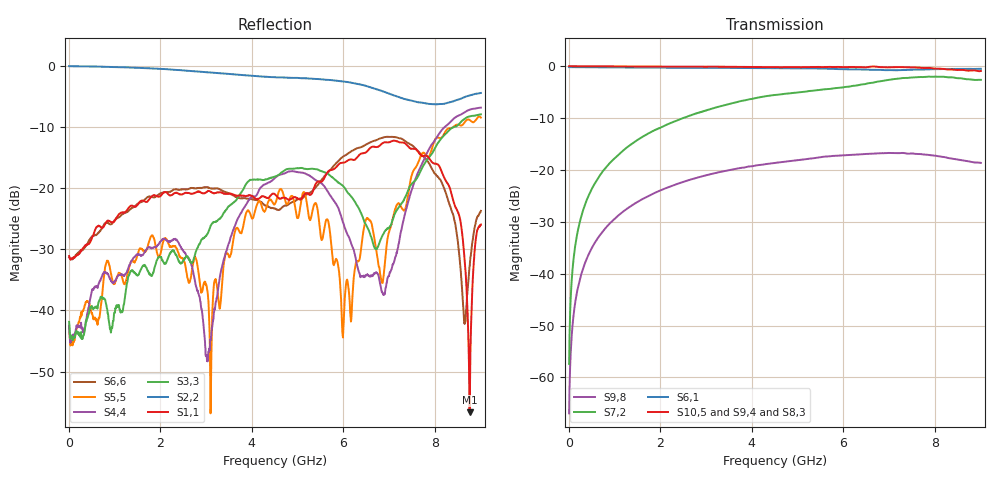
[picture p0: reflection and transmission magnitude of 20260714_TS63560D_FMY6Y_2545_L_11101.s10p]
# GHz S DB R 50
! CMT, SN0916, 25263762, 26.7.0
! Date: 15.07.2026 13:50:19
! Data: Format
! Freq S1.1:dB/Ang S1.2:dB/Ang S1.3:dB/Ang S1.4:dB/Ang S1.5:dB/Ang S1.6:dB/Ang S1.7:dB/Ang S1.8:dB/Ang S1.9:dB/Ang S1.10:dB/Ang
!  S2.1:dB/Ang S2.2:dB/Ang S2.3:dB/Ang S2.4:dB/Ang S2.5:dB/Ang S2.6:dB/Ang S2.7:dB/Ang S2.8:dB/Ang S2.9:dB/Ang S2.10:dB/Ang
!  S3.1:dB/Ang S3.2:dB/Ang S3.3:dB/Ang S3.4:dB/Ang S3.5:dB/Ang S3.6:dB/Ang S3.7:dB/Ang S3.8:dB/Ang S3.9:dB/Ang S3.10:dB/Ang
!  S4.1:dB/Ang S4.2:dB/Ang S4.3:dB/Ang S4.4:dB/Ang S4.5:dB/Ang S4.6:dB/Ang S4.7:dB/Ang S4.8:dB/Ang S4.9:dB/Ang S4.10:dB/Ang
!  S5.1:dB/Ang S5.2:dB/Ang S5.3:dB/Ang S5.4:dB/Ang S5.5:dB/Ang S5.6:dB/Ang S5.7:dB/Ang S5.8:dB/Ang S5.9:dB/Ang S5.10:dB/Ang
!  S6.1:dB/Ang S6.2:dB/Ang S6.3:dB/Ang S6.4:dB/Ang S6.5:dB/Ang S6.6:dB/Ang S6.7:dB/Ang S6.8:dB/Ang S6.9:dB/Ang S6.10:dB/Ang
!  S7.1:dB/Ang S7.2:dB/Ang S7.3:dB/Ang S7.4:dB/Ang S7.5:dB/Ang S7.6:dB/Ang S7.7:dB/Ang S7.8:dB/Ang S7.9:dB/Ang S7.10:dB/Ang
!  S8.1:dB/Ang S8.2:dB/Ang S8.3:dB/Ang S8.4:dB/Ang S8.5:dB/Ang S8.6:dB/Ang S8.7:dB/Ang S8.8:dB/Ang S8.9:dB/Ang S8.10:dB/Ang
!  S9.1:dB/Ang S9.2:dB/Ang S9.3:dB/Ang S9.4:dB/Ang S9.5:dB/Ang S9.6:dB/Ang S9.7:dB/Ang S9.8:dB/Ang S9.9:dB/Ang S9.10:dB/Ang
!  S10.1:dB/Ang S10.2:dB/Ang S10.3:dB/Ang S10.4:dB/Ang S10.5:dB/Ang S10.6:dB/Ang S10.7:dB/Ang S10.8:dB/Ang S10.9:dB/Ang S10.10:dB/Ang
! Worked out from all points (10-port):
!   2001 points, 10 MHz to 9 GHz, reference 50 ohm
!   strongest paths, dB at 10 MHz, 2.257 GHz, 4.505 GHz, 6.753 GHz, 9 GHz:
!     S10,5: -0.1, -0.2, -0.2, -0.2, -1.0
!     S9,4: -0.1, -0.2, -0.4, -0.4, -1.5
!     S8,3: -0.1, -0.2, -0.4, -0.4, -1.3
!     S6,1: -0.3, -0.4, -0.5, -0.8, -0.6
!     S7,2: -57.4, -10.9, -5.6, -3.0, -2.7
!     S9,8: -66.9, -23.1, -18.7, -16.9, -18.7
!   lowest |S11| = -56.7 dB at 8.753 GHz (marker M1), VSWR 1.00, Z = 50 - j0.145 ohm
!   |S11| at or under -10 dB: start of sweep to end of sweep
